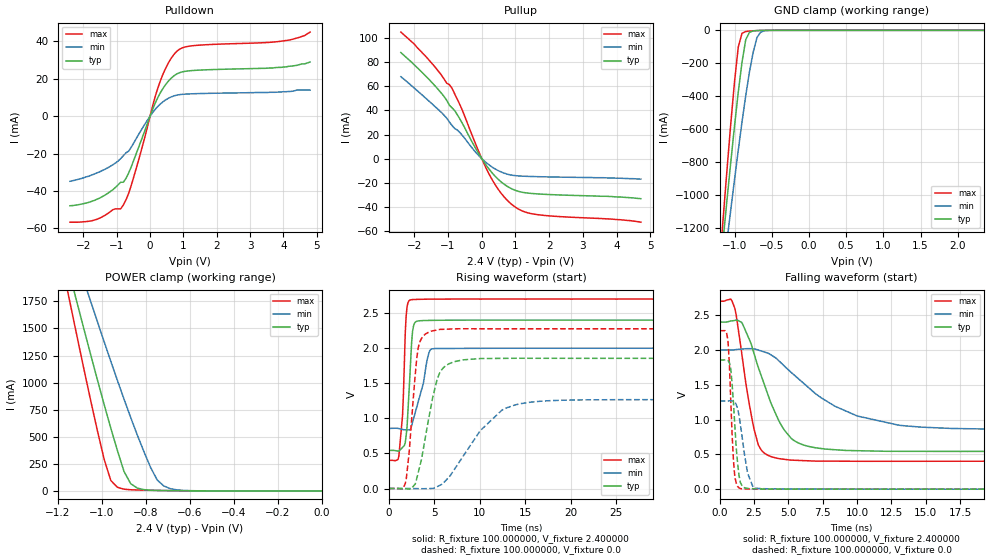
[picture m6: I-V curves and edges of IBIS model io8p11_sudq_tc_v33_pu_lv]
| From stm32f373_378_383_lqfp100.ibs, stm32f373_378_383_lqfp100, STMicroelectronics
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|   Model io8p11_sudq_tc_v33_pu_lv
[Model]  io8p11_sudq_tc_v33_pu_lv
Model_type I/O
Polarity   Non-Inverting
Enable   Active-Low
Vinl =   0.720000V
Vinh =   1.680000V
Vmeas =  1.200000V
Cref =   50.000000pF
Rref =   100.000000M
Vref =   0.0V
C_comp   1.373400pF   1.288200pF   1.481900pF
[Temperature Range]   25.000000   0.125000k   -40.000000
[Pullup Reference]   2.400000V   2.000000V   2.700000V
[Pulldown Reference]   0.0V   0.0V   0.0V
[POWER Clamp Reference]   2.400000V   2.000000V   2.700000V
[GND Clamp Reference]   0.0V   0.0V   0.0V
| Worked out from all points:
|   slope of the pulldown table from 0 to 0.36 V, typ, clamps not added: 25.7 ohm
|   slope of the pullup table from 0 to 0.36 V, typ, clamps not added: 26.8 ohm
|   GND clamp passes 1 mA (typ) near -0.67 V on its own axis
|   POWER clamp passes 1 mA (typ) near -0.60 V on its own axis
|   rising waveform, R_fixture 100.000000, V_fixture 2.400000: 20-80 % time 465ps typ, 1.21ns min, 432ps max; typ from 0.543 V to 2.4 V
|   rising waveform, R_fixture 100.000000, V_fixture 0.0: 20-80 % time 1.67ns typ, 4.48ns min, 863ps max; typ from 0.001 V to 1.86 V
|   falling waveform, R_fixture 100.000000, V_fixture 2.400000: 20-80 % time 2.12ns typ, 4.93ns min, 1.11ns max; typ from 2.4 V to 0.543 V
|   falling waveform, R_fixture 100.000000, V_fixture 0.0: 20-80 % time 393ps typ, 574ps min, 291ps max; typ from 1.86 V to 0.001 V
[Pulldown]
|Voltage   I(typ)   I(min)   I(max)
-2.4V     -47.9mA    -34.8mA    -56.7mA
-1.6V     -44.5mA    -30.4mA    -55.2mA
-880mV    -35.33mA   -22.63mA   -49.55mA
-800mV    -35.33mA   -21.13mA   -47.42mA
-640mV    -30.33mA   -18.65mA   -41.16mA
-480mV    -23.12mA   -14mA      -31.94mA
240mV     10.22mA    5.339mA    15.38mA
480mV     17.22mA    8.864mA    26.1mA
800mV     22.59mA    11.27mA    34.68mA
1.28V     24.44mA    12mA       37.7mA
4.16V     26.7mA     13.2mA     40.7mA
4.8V      29mA       14mA       45mA
[Pullup]
|Voltage   I(typ)   I(min)   I(max)
-2.4V     88mA       68mA       105mA
-2V       77.8mA     58.5mA     95mA
-1.36V    59.6mA     42.5mA     75.1mA
-880mV    42.12mA    27.44mA    58.22mA
-560mV    28.45mA    18.75mA    39mA
-160mV    7.44mA     4.66mA     10.64mA
160mV     -6.607mA   -3.947mA   -9.704mA
480mV     -16.91mA   -9.806mA   -25.1mA
880mV     -24.89mA   -13.63mA   -37.75mA
1.2V      -27.87mA   -14.5mA    -43.37mA
1.6V      -29.13mA   -14.89mA   -46.24mA
4.72V     -33.2mA    -17mA      -52.7mA
[GND_clamp]
|Voltage   I(typ)   I(min)   I(max)
-2.4V     -7.358A    -6.372A    -8.78A
-1.2V     -1.489A    -1.65A     -1.416A
-1.15V    -1.254A    -1.461A    -1.124A
-1.1V     -1.024A    -1.273A    -838.2mA
-1.05V    -797.6mA   -1.088A    -563.1mA
-950mV    -374.6mA   -728.7mA   -100.8mA
-900mV    -194.3mA   -557.9mA   -18.01mA
-850mV    -56.94mA   -397.4mA   -7.08mA
-750mV    -3.582mA   -133.8mA   -2.771mA
-700mV    -1.516mA   -44.7mA    -1.516mA
-600mV    -235.4uA   -2.939mA   -209.5uA
2.35V     0A         0A         0A
[POWER_clamp]
|Voltage   I(typ)   I(min)   I(max)
-2.4V     9.979A     9.967A     9.901A
-1.17V    2.182A     2.481A     1.978A
-1.14V    1.945A     2.294A     1.683A
-1.11V    1.71A      2.108A     1.391A
-1.08V    1.476A     1.923A     1.102A
-1.05V    1.245A     1.739A     819.9mA
-960mV    578.3mA    1.196A     96.08mA
-900mV    179.5mA    846.7mA    16.05mA
-870mV    67.19mA    678.8mA    10.83mA
-780mV    6.763mA    219.9mA    5.868mA
-720mV    3.368mA    46.35mA    3.823mA
0V        0A         0A         0A
[Ramp]
| variable   typ   min   max
dV/dt_r  1.11279/1.66590n   0.75936/4.47595n   1.36532/0.85756n
dV/dt_f  1.11422/2.11945n   0.68574/4.92144n   1.37889/1.10675n
R_load = 100.000000
[Rising Waveform]
R_fixture= 100.000000
V_fixture= 2.400000
V_fixture_min= 2.000000
V_fixture_max= 2.700000
|time   V(typ)   V(min)   V(max)
0s        543.1mV    857mV      401.7mV
1.101ns   533mV      854.7mV    461.7mV
1.502ns   586mV      842.1mV    1.034V
1.902ns   757.8mV    836.8mV    2.463V
2.302ns   1.58V      835.7mV    2.685V
2.603ns   2.237V     944.5mV    2.692V
2.803ns   2.351V     1.038V     2.694V
4.404ns   2.396V     1.934V     2.699V
4.805ns   2.397V     1.991V     2.699V
49.85ns   2.4V       2V         2.7V
[Rising Waveform]
R_fixture= 100.000000
V_fixture= 0.0
V_fixture_min= 0.0
V_fixture_max= 0.0
|time   V(typ)   V(min)   V(max)
0s        956.5uV    1.197mV    860.5uV
1.802ns   -2.083mV   1.234mV    70.44mV
2.202ns   -6.517mV   1.093mV    478.8mV
3.203ns   215.1mV    -1.113mV   1.986V
4.605ns   1.152V     1.174mV    2.241V
5.305ns   1.555V     27.11mV    2.26V
6.406ns   1.763V     135.6mV    2.271V
10.01ns   1.851V     818.9mV    2.276V
14.11ns   1.856V     1.199V     2.276V
49.85ns   1.856V     1.267V     2.276V
[Falling Waveform]
R_fixture= 100.000000
V_fixture= 2.400000
V_fixture_min= 2.000000
V_fixture_max= 2.700000
|time   V(typ)   V(min)   V(max)
0s        2.4V       2V         2.7V
1.101ns   2.424V     2.003V     2.597V
1.702ns   2.357V     2.014V     1.81V
2.202ns   2.129V     2.018V     1.169V
2.803ns   1.753V     1.999V     640.6mV
4.204ns   1.026V     1.863V     443.7mV
6.306ns   623.3mV    1.487V     409.2mV
10.01ns   553.3mV    1.052V     401.6mV
13.11ns   544.4mV    917.7mV    401.5mV
49.85ns   543.1mV    857mV      401.7mV
[Falling Waveform]
R_fixture= 100.000000
V_fixture= 0.0
V_fixture_min= 0.0
V_fixture_max= 0.0
|time   V(typ)   V(min)   V(max)
0s        1.856V     1.267V     2.276V
600.6ps   1.852V     1.268V     2.137V
800.8ps   1.734V     1.271V     1.303V
1.001ns   1.245V     1.265V     413.2mV
1.101ns   917.1mV    1.252V     176.8mV
1.301ns   379mV      1.156V     42.4mV
1.502ns   98.49mV    935.6mV    10.09mV
2.002ns   13.19mV    264.1mV    3.025mV
2.803ns   3.913mV    11.47mV    1.844mV
49.85ns   956.5uV    1.197mV    860.5uV
